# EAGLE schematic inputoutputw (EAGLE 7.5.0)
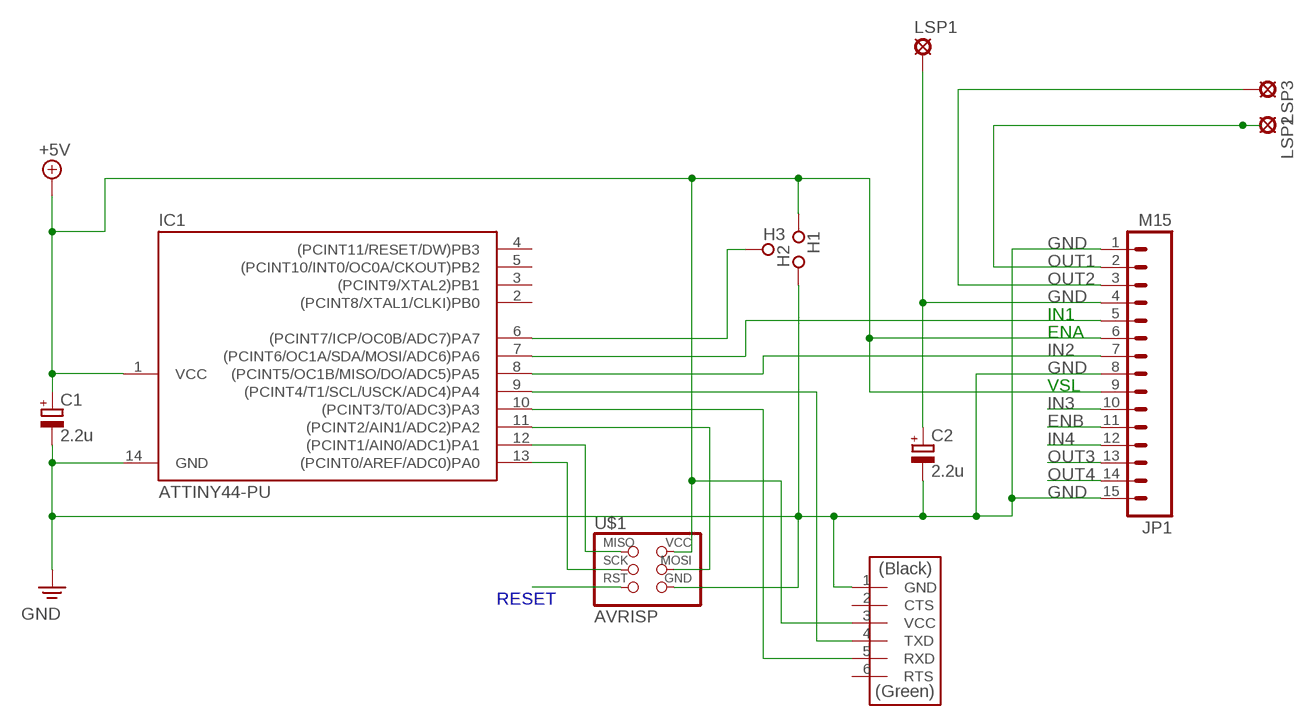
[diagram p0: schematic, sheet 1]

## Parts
C1  2.2u  CPOL-EUC/6032-28R  [C/6032-28R]
C2  2.2u  CPOL-EUC/6032-28R  [C/6032-28R]
H1  SPECIAL_DRILL_0.1800  [PAD_0.1800]
H2  SPECIAL_DRILL_0.1800  [PAD_0.1800]
H3  SPECIAL_DRILL_0.1800  [PAD_0.1800]
IC1  ATTINY44-PU  [DIL14]
JP1  M15  [1X15]
LSP1  LSP13  [LSP13]
LSP2  LSP13  [LSP13]
LSP3  LSP13  [LSP13]
U$1  AVRISP  [2X03]
U$2  FTDI-SMD-HEADER  [1X06SMD]

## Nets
+5V: C1.+ H1.1 IC1.1(VCC) JP1.6 JP1.9 U$1.2(VCC) U$2.3(VCC)
ENB: JP1.11
GND: C1.- C2.- H2.1 IC1.14(GND) JP1.1 JP1.8 JP1.15 U$1.6(GND) U$2.1(GND)
IN2: IC1.8((PCINT5/OC1B/MISO/DO/ADC5)PA5) JP1.7
IN3: JP1.10
IN4: JP1.12
N$1: IC1.7((PCINT6/OC1A/SDA/MOSI/ADC6)PA6) JP1.5
N$2: C2.+ JP1.4 LSP1.MP
N$3: H3.1 IC1.6((PCINT7/ICP/OC0B/ADC7)PA7)
N$4: U$1.5(RST)
N$5: IC1.13((PCINT0/AREF/ADC0)PA0) U$1.3(SCK)
N$6: IC1.12((PCINT1/AIN0/ADC1)PA1) U$1.1(MISO)
N$7: IC1.11((PCINT2/AIN1/ADC2)PA2) U$1.4(MOSI)
N$8: IC1.9((PCINT4/T1/SCL/USCK/ADC4)PA4) U$2.4(TXD)
N$9: IC1.10((PCINT3/T0/ADC3)PA3) U$2.5(RXD)
OUT1: JP1.2 LSP2.MP
OUT2: JP1.3 LSP3.MP
OUT3: JP1.13
OUT4: JP1.14
Unconnected: IC1.2((PCINT8/XTAL1/CLKI)PB0) IC1.3((PCINT9/XTAL2)PB1) IC1.4((PCINT11/RESET/DW)PB3) IC1.5((PCINT10/INT0/OC0A/CKOUT)PB2) U$2.2(CTS) U$2.6(RTS)

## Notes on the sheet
- IN1
- ENA
- VSL
- RESET

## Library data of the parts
C1 C2 = rcl:CPOL-EU: POLARIZED CAPACITOR, European symbol
H1-H3 = special-drill:SPECIAL_DRILL_: Special drills
IC1 = fab:ATTINY44
JP1 = SparkFun:M15: Header 15 Standard 15-pin 0.1" header. Use with straight break away headers (SKU : PRT-00116), right angle break away headers (PRT-00553), swiss pins (PRT-00743), machine pins (PRT-00117), and female headers (PRT-00115).
LSP1-LSP3 = solpad:LSP13: SOLDER PAD
U$1 = fab:AVRISP
U$2 = fab:FTDI-SMD-HEADER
